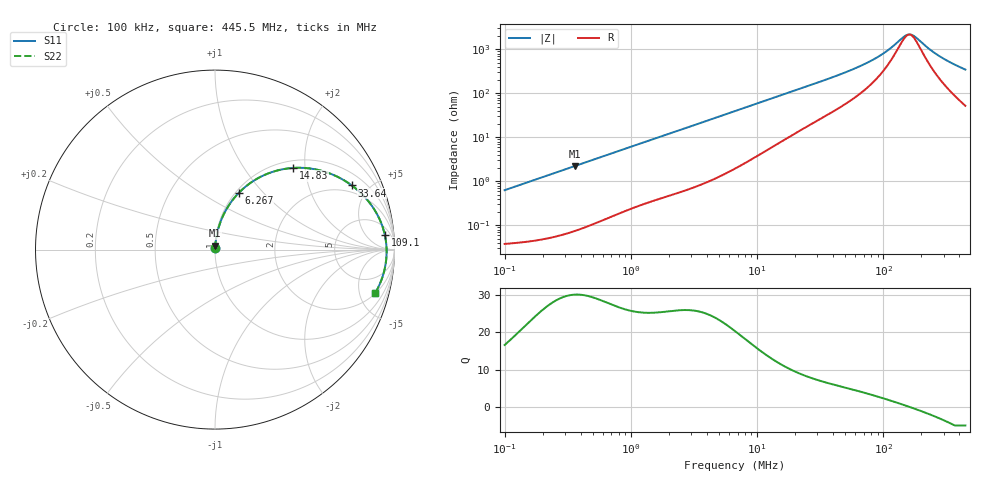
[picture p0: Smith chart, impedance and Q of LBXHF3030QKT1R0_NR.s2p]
! LBXHF3030QKT1R0_NR  S-PARAMETER MODEL  ( General Type )
! Model Generated by TAIYO YUDEN Corporation (http://www.ty-top.com)
! Version 1.0
! TAIYO YUDEN Control No. 210113NI43SB-FBB
! Copyright(c) 2021 TAIYO YUDEN CO.,LTD. All Rights Reserved.
! Product Description (link to TY-COMPAS)
! https://ds.yuden.co.jp/TYCOMPAS/or/detail?pn=LBXHF3030QKT1R0MNR&u=M
! Products Name : Inductors
! Characteristics :
!  Inductance : 1.0 uH , SRF(min) : 100 MHz , DC Resistance(max) : 0.033 Ohm
!  Rated Current : Saturation :2300 mA , Temp Rise : 1700 mA
!  Case Size : 3.0 x 3.0 / 0.118 x 0.118 [mm/inch] , Thickness : 1.5 / 0.059 [mm/inch]
!  (Conditions: Temperature = 25 degC , DC Bias Current/Voltage = 0A / 0V)
! External Node Assignments :
!  1  o---GGG---o  2
! GND o---------o GND
! Frequency Range : 0.1MHz  -  445.549718MHz  [ 402 STEP ]
# MHz S RI R 50
! Freq[MHz].  S11 Real  S11 Imag  S21 Real  S21 Imag  S12 Real  S12 Imag  S22 Real  S22 Imag
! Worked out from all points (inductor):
!   401 points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, 100 kHz to 445.5 MHz, reference 50 ohm
!   read as one part in series: L = 1 uH near 104.3 kHz
!   highest Q = 30.1 at 360.1 kHz (marker M1), where L = 994 nH
!   self-resonance near 160 MHz
!   S11 on the Smith chart (normalised r, x): 100 kHz: 1.00, +0.01; 6.267 MHz: 1.04, +0.74; 14.83 MHz: 1.15, +1.74; 33.64 MHz: 1.58, +3.88; 109.1 MHz: 10, +17; 445.5 MHz: 2.04, -6.84
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0.1  0.000419 0.00629  0.9996 -0.00629  0.9996 -0.00629  0.000419 0.00629
0.360128  0.00125 0.0224  0.9987 -0.0224  0.9987 -0.0224  0.00125 0.0224
0.408498  0.00149 0.0254  0.9985 -0.0254  0.9985 -0.0254  0.00149 0.0254
1.668708  0.0139 0.099  0.9861 -0.099  0.9861 -0.099  0.0139 0.099
3.629971  0.052 0.2033  0.948 -0.2033  0.948 -0.2033  0.052 0.2033
6.267313  0.1329 0.3165  0.8671 -0.3165  0.8671 -0.3165  0.1329 0.3165
6.81664  0.1524 0.3354  0.8476 -0.3354  0.8476 -0.3354  0.1524 0.3354
9.742006  0.2617 0.4093  0.7383 -0.4093  0.7383 -0.4093  0.2617 0.4093
14.82836  0.4367 0.4552  0.5633 -0.4552  0.5633 -0.4552  0.4367 0.4552
27.26705  0.6933 0.4004  0.3067 -0.4004  0.3067 -0.4004  0.6933 0.4004
33.64036  0.7624 0.3574  0.2376 -0.3574  0.2376 -0.3574  0.7624 0.3574
67.28132  0.9054 0.1927  0.0946 -0.1927  0.0946 -0.1927  0.9054 0.1927
88.40639  0.9329 0.1293  0.0671 -0.1293  0.0671 -0.1293  0.9329 0.1293
109.0702  0.9461 0.0825  0.0539 -0.0825  0.0539 -0.0825  0.9461 0.0825
111.3854  0.947 0.0779  0.053 -0.0779  0.053 -0.0779  0.947 0.0779
146.3583  0.9552 0.019  0.0448 -0.019  0.0448 -0.019  0.9552 0.019
155.8778  0.9559 0.00557  0.0441 -0.00557  0.0441 -0.00557  0.9559 0.00557
166.0164  0.9562 -0.00793  0.0438 0.00793  0.0438 0.00793  0.9562 -0.00793
180.5676  0.9559 -0.026  0.0441 0.026  0.0441 0.026  0.9559 -0.026
227.5016  0.9512 -0.0769  0.0488 0.0769  0.0488 0.0769  0.9512 -0.0769
274.843  0.9424 -0.1206  0.0576 0.1206  0.0576 0.1206  0.9424 -0.1206
445.5497  0.8916 -0.2441  0.1084 0.2441  0.1084 0.2441  0.8916 -0.2441
